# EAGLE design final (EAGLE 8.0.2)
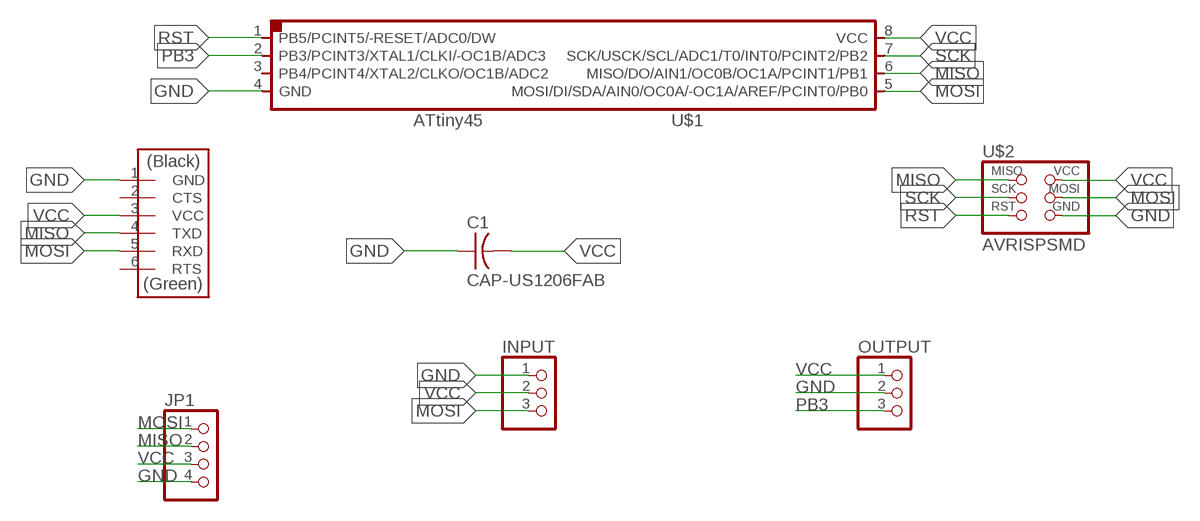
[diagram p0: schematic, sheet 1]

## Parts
C1  CAP-US1206FAB  [C1206FAB]
INPUT  PINHD-1X3  [1X03]
JP1  PINHD-1X4  [1X04]
OUTPUT  PINHD-1X3  [1X03]
U$1  ATTINY45SI  [SOIC8]
U$2  AVRISPSMD  [2X03SMD]
U$3  FTDI-SMD-HEADER  [1X06SMD]

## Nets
GND: C1.1 INPUT.1 JP1.4 OUTPUT.2 U$1.4(GND) U$2.6(GND) U$3.1(GND)
MISO: JP1.2 U$1.6(MISO/DO/AIN1/OC0B/OC1A/PCINT1/PB1) U$2.1(MISO) U$3.4(TXD)
MOSI: INPUT.3 JP1.1 U$1.5(MOSI/DI/SDA/AIN0/OC0A/-OC1A/AREF/PCINT0/PB0) U$2.4(MOSI) U$3.5(RXD)
PB3: OUTPUT.3 U$1.2(PB3/PCINT3/XTAL1/CLKI/-OC1B/ADC3)
RST: U$1.1(PB5/PCINT5/-RESET/ADC0/DW) U$2.5(RST)
SCK: U$1.7(SCK/USCK/SCL/ADC1/T0/INT0/PCINT2/PB2) U$2.3(SCK)
VCC: C1.2 INPUT.2 JP1.3 OUTPUT.1 U$1.8(VCC) U$2.2(VCC) U$3.3(VCC)
Unconnected: U$1.3(PB4/PCINT4/XTAL2/CLKO/OC1B/ADC2) U$3.2(CTS) U$3.6(RTS)

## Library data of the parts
C1 = fab (1):CAP-US
INPUT OUTPUT = pinhead:PINHD-1X3: PIN HEADER
JP1 = pinhead:PINHD-1X4: PIN HEADER
U$1 = fab (1):ATTINY45
U$2 = fab (1):AVRISP
U$3 = fab (1):FTDI-SMD-HEADER

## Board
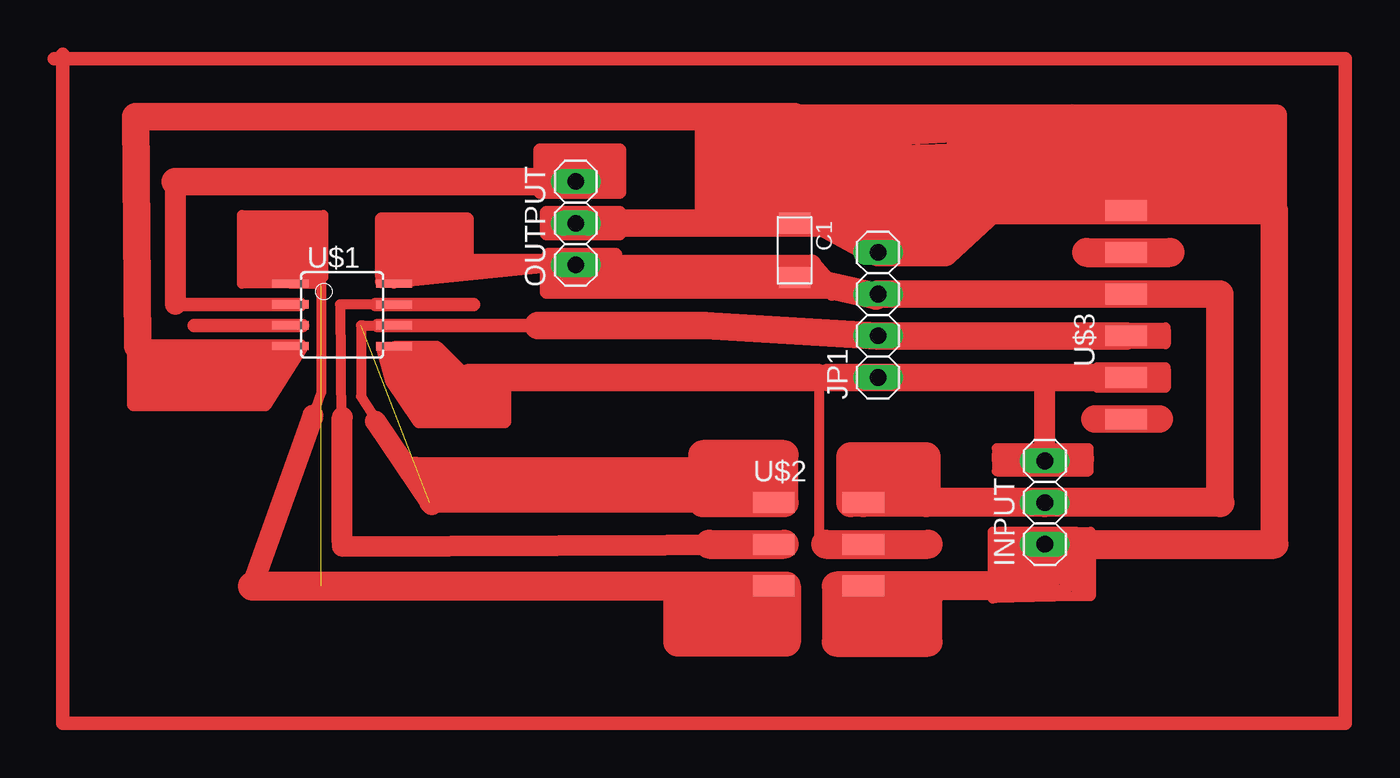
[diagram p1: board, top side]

No outline drawn. Coordinates in mm, seen from the top.
Copper layers (1*16): Top 0.035mm / dielectric 1.5mm / Bottom 0.035mm
Design rules "default *": minimum track width 20mil, minimum drill 16mil, track to track 16mil, track to pad 16mil, pad to pad 16mil, via to via 8mil, smd to smd 8mil, copper to edge 20mil, drill to drill 8mil, minimum pad ring 10mil, minimum via ring 8mil, stop-mask expansion 4mil, vias tented up to drill 0mil, thermal gap 10mil

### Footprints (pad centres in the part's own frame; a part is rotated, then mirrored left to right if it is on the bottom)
C1206FAB = smd 1.27 x 1.905: 1 -1.651,0; 2 1.651,0
1X03 = drill 1.016 long: 1 -2.54,0; 2 0,0; 3 2.54,0
1X04 = drill 1.016 long: 1 -3.81,0; 2 -1.27,0; 3 1.27,0; 4 3.81,0
SOIC8 = smd 0.5 x 2.2: 1 -1.905,-3.154; 2 -0.645,-3.154; 3 0.625,-3.154; 4 1.895,-3.154; 5 1.905,3.154; 6 0.635,3.154; 7 -0.635,3.154; 8 -1.905,3.154
2X03SMD = smd 2.54 x 1.27: 1 -2.54,2.54; 2 2.92,2.54; 3 -2.54,0; 4 2.92,0; 5 -2.54,-2.54; 6 2.92,-2.54
1X06SMD = smd 2.54 x 1.27: 1 0,6.35; 2 0,3.81; 3 0,1.27; 4 0,-1.27; 5 0,-3.81; 6 0,-6.35

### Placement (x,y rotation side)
C1  67.31,39.5 270 top
INPUT  82.55,24.13 90 top
JP1  72.39,35.56 90 top
OUTPUT  53.98,41.15 90 top
U$1  39.75,35.56 270 top
U$2  68.58,21.59 0 top
U$3  87.5,35.56 0 top

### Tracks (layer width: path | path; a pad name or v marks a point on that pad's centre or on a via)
GND
  Top 0.61: 27.3,33.66 30.72,33.66 U$1.4
  Top 1.676: 96.52,21.59 96.52,41.91 U$3.1 79.25,41.91 76.45,39.37 JP1.4 69.09,41.15 C1.1 | 27.3,33.66 27.18,47.62 67.31,47.62 C1.1 | OUTPUT.2 C1.1
  Top 1.778: 75.06,19.05 82.55,19.05 INPUT.1 96.52,21.59 | 75.06,19.05 U$2.6 | 75.06,19.05 69.85,19.05 69.85,15.62 75.44,15.62 75.44,18.29 71.37,17.91 71.25,16.89 74.42,17.27
MISO  (1 unrouted)
  Top 0.61: 61.85,34.92 61.59,34.92 54.36,34.92 51.69,34.92 49.28,34.92 U$1.6 41.91,34.92 41.02,34.92 | 40.89,34.92 41.02,34.92 | 41.02,34.92 40.89,34.92 | 40.89,34.92 40.89,30.61 45.09,24.13
  Top 0.813: 41.91,34.92 49.28,34.92 51.69,34.92 54.36,34.92 61.59,34.92 62.48,34.92
  Top 1.27: U$2.1 61.98,24.13 61.72,24.13 45.09,24.13
  Top 1.676: 61.85,34.92 JP1.2 U$3.4 | 61.59,34.92 51.69,34.92
  Top 1.778: 61.98,24.13 66.67,24.13 66.67,27.05 61.72,27.05 61.72,24.13 63.25,25.78 65.15,25.65
MOSI
  Top 0.61: U$1.5 45.59,33.66 47.5,31.75 | 70.23,21.59 U$2.4 69.22,21.59 68.83,21.59 68.83,31.62 68.71,31.75 69.34,31.75 69.09,31.5
  Top 1.27: INPUT.3 82.55,31.75
  Top 1.676: 69.34,31.75 JP1.1 82.55,31.75 U$3.5 | 68.71,31.75 47.5,31.75
  Top 1.778: 69.22,21.59 75.44,21.59
N$1
  Top 0.813: 37.21,36.2 29.72,36.2
N$2
  Top 0.813: 37.34,34.92 30.73,34.92
N$3
  Top 0.813: 37.21,33.66 27.05,33.66 27.05,30.1 35.05,30.1 37.21,33.53 27.56,33.02 27.43,30.61 34.92,30.73 36.2,32.89 27.81,32.51 28.19,31.24 34.92,31.37 35.31,32.38 27.94,32 35.05,31.88
N$4
  Top 0.813: 47.37,31.62 45.21,33.4 42.29,33.4 42.8,31.5 | 42.8,31.5 47.5,31.5 42.93,32 43.05,32.77 45.21,32.64 46.35,32.13 43.69,32.26 42.8,31.5 | 42.8,31.5 44.45,29.08 49.66,29.08 49.66,31.11 43.69,31.11 44.96,29.59 49.28,29.59 49.15,30.61 44.45,30.61 45.34,30.1 48.9,30.23
N$5
  Top 0.813: 42.16,37.59 53.98,38.86 47.37,38.86 | 47.37,38.86 42.16,38.86 | 42.16,38.86 42.16,38.48 | 42.16,38.48 42.16,37.97 46.23,38.35 42.29,38.35 42.16,38.48 | 42.16,38.86 42.16,41.4 47.37,41.4 47.37,38.86 | 47.37,38.86 42.67,39.37 42.67,40.77 46.86,40.77 46.86,39.37 43.18,39.88 43.05,40.26 46.61,40.01
N$6
  Top 1.27: 39.75,21.72 39.75,29.34
N$7
  Top 1.27: 45.21,24 41.78,29.08
N$8
  Top 1.27: 37.97,29.46 34.29,19.18
N$9
  Top 1.778: 62.1,21.59 66.67,21.59
N$10
  Top 1.778: 44.96,24.89 61.59,24.89
N$11
  Top 1.778: 44.2,26.04 62.1,26.04
N$12
  Top 1.778: 85.09,39.37 90.17,39.37
N$13
  Top 0.813: 52.32,39.12 52.32,39.24 56.39,39.24 56.39,36.96 | 56.39,36.96 52.2,36.96 52.2,38.23 55.88,38.1 55.88,37.59 52.83,37.59 | 56.39,36.96 70.23,36.96 65.91,37.72 56.9,37.59
N$14
  Top 0.813: 56.64,41.78 52.2,41.78 52.2,40.51 56.64,40.51
N$15
  Top 0.813: 51.82,43.05 56.64,43.05 56.64,45.59 51.82,45.59 51.82,44.58 52.7,45.09 56.13,45.09 56.13,43.69 54.86,43.69 55.75,44.45 52.45,44.45
N$16
  Top 0.813: 68.45,38.73 69.34,37.72
N$17
  Top 0.813: 69.6,36.96 69.6,36.83
N$18
  Top 0.813: 67.82,40.77 78.61,40.89 75.69,40.39 72.01,40.26
N$19
  Top 1.27: 62.87,42.16 81.28,42.16 75.56,41.15 70.1,41.4 62.99,41.53 62.99,46.99 61.85,47.5 61.85,41.66 63.75,46.61 66.29,46.48 66.55,43.18 63.5,42.8 64.26,45.59 65.53,45.85 66.17,43.94 64.39,43.69 65.02,44.83 67.44,47.75 84.2,47.75 | 84.2,47.75 96.65,47.75 96.65,41.4 95.76,46.74 84.2,47.75 | 84.2,47.75 68.33,47.12 68.45,43.18 92.84,43.31 95.5,43.18 95,45.97 82.17,46.99 69.22,46.23 69.22,44.45 70.36,44.07 94.74,44.2 94.61,45.09 69.72,44.7 69.85,45.21 90.42,45.72 77.22,46.1
N$20
  Top 0.61: 87,34.8 89.92,34.8
N$21
  Top 0.61: 89.92,34.67 89.92,33.78 87.5,33.78 89.79,34.29 88.65,34.42
N$22
  Top 0.61: 87.25,32.26 89.92,32.26 89.92,31.11 85.72,31.11 85.72,32.38 89.92,32.38
N$23
  Top 0.61: 88.65,32 89.53,31.75 89.53,31.62 88.65,31.62
N$24
  Top 1.676: 85.6,29.21 89.53,29.21
N$25
  Top 1.676: 80.14,26.8 84.71,26.8
N$26
  Top 0.61: 79.63,27.05 79.63,26.92 79.63,26.04 85.22,26.04 85.22,27.43 79.63,27.43 79.63,27.05
N$27
  Top 0.61: 84.45,22.35 80.26,22.35 | 80.26,22.35 79.76,22.35 | 79.76,22.35 79.63,19.68 79.38,19.68 79.38,22.35 79.76,22.35 | 80.26,22.35 80.01,19.94 81.66,20.07 81.66,21.97 80.64,21.97 80.52,20.19 81.41,20.45 81.28,21.84 81.03,20.57 84.45,22.35 | 84.45,22.35 84.45,18.41 | 84.45,18.41 79.38,18.29 83.95,18.92 84.07,20.57 83.57,20.57 83.69,19.3 | 84.45,22.35 85.34,22.35 85.34,18.41 84.45,18.41 | 84.45,18.41 84.84,18.67 84.84,20.57
N$28
  Top 0.813: 22.23,51.18 100.84,51.18 100.84,10.67 22.73,10.67 22.73,51.44
PB3
  Top 0.61: 29.59,36.2 U$1.2
  Top 1.27: 29.59,43.69 29.59,36.2
  Top 1.676: OUTPUT.3 29.59,43.69
RST  (1 unrouted)
  Top 0.61: U$1.1 37.21,37.47 | 37.21,37.47 38.48,37.47 38.48,30.86 34.29,19.05 | 38.48,19.05 38.86,19.05 | 37.21,37.47 33.66,37.47 33.66,41.66 38.61,41.66 38.61,37.85 34.16,37.97 34.16,41.15 38.23,41.15 38.1,38.35 34.42,38.35 34.42,40.64 37.72,40.64 37.59,38.61 37.08,38.61 | 37.08,38.61 34.8,38.61 34.67,40.26 37.34,40.13 37.08,38.61 | 37.08,38.61 35.05,39.24 35.18,39.75 37.08,39.88 36.83,38.99 35.31,39.5 36.83,39.24
  Top 1.778: 61.85,19.05 38.86,19.05 34.29,19.05 | 61.85,19.05 U$2.5 | 61.85,19.05 66.8,19.05 66.8,15.62 60.2,15.62 60.2,18.67 65.41,17.91 65.91,16.89 61.34,17.02
SCK
  Top 0.61: U$1.7 41.78,36.2 39.62,36.2 39.75,21.46
  Top 0.813: 41.78,36.2 47.75,36.2
  Top 1.27: 39.75,21.46 U$2.3
VCC
  Top 0.61: JP1.3 72.26,36.7 | OUTPUT.1 U$1.8 42.8,37.57 | C1.2 68.33,38.61
  Top 1.27: OUTPUT.1 68.33,38.61
  Top 1.676: 93.22,24.13 93.22,36.83 U$3.3 JP1.3 | C1.2 72.26,36.7
  Top 1.778: 75.31,24.13 INPUT.2 93.22,24.13 | 75.31,24.13 U$2.2 | 75.31,24.13 70.74,24.13 70.74,26.92 75.31,26.92 75.31,24.77 74.55,25.53 72.01,25.53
